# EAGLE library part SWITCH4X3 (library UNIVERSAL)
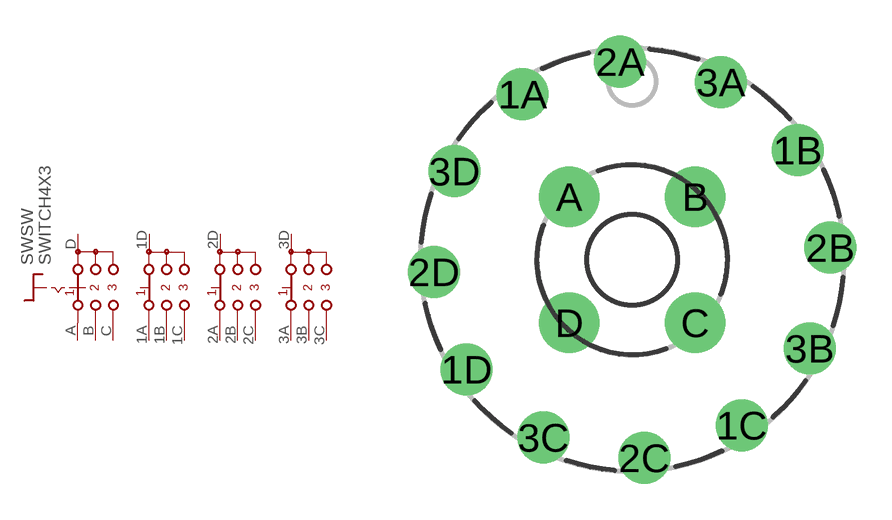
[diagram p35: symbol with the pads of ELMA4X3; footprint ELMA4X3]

Designator prefix SW; gates SW=SWITCH4X3 G$2=SWITCH4X3B G$3=SWITCH4X3B G$4=SWITCH4X3B

## SWITCH4X3  [ELMA4X3]
1A  G$2:B1  pas
1B  G$2:B2  pas
1C  G$2:B3  pas
1D  G$2:B  pas
2A  G$3:B1  pas
2B  G$3:B2  pas
2C  G$3:B3  pas
2D  G$3:B  pas
3A  G$4:B1  pas
3B  G$4:B2  pas
3C  G$4:B3  pas
3D  G$4:B  pas
A  SW:A1  pas
B  SW:A2  pas
C  SW:A3  pas
D  SW:A  pas

## Footprint ELMA4X3 (pad centres in mm)
drill 1.3 pad 2.184: 1A -4.609,6.963; 1B 6.963,4.609; 1C 4.609,-6.963; 1D -6.963,-4.609; 2A -0.51,8.334; 2B 8.334,0.51; 2C 0.51,-8.334; 2D -8.334,-0.51; 3A 3.726,7.473; 3B 7.473,-3.726; 3C -3.726,-7.473; 3D -7.473,3.726
drill 1.5 pad 2.54: A -2.652,2.652; B 2.652,2.652; C 2.652,-2.652; D -2.652,-2.652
